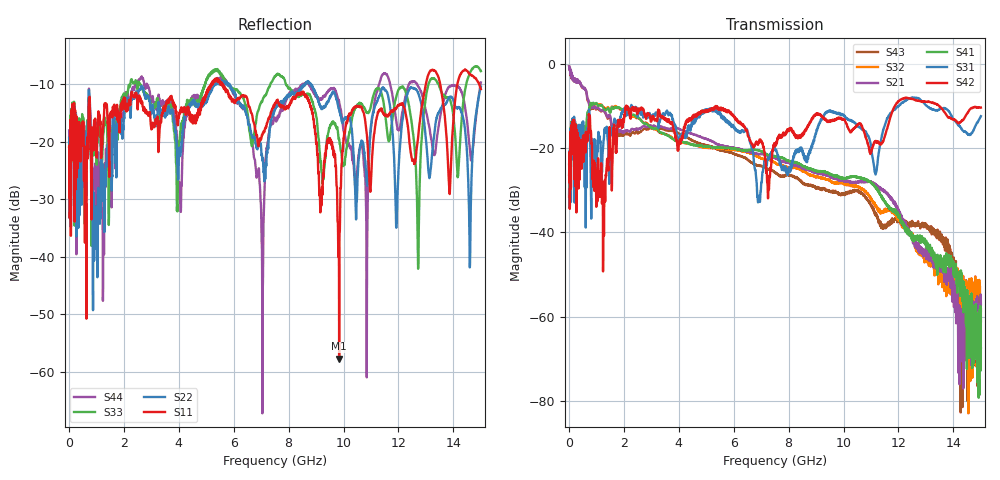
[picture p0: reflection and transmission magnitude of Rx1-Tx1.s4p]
! FILE: N:\QM 2007\Prüfprotokolle\Highspeed\Konfektionierte Ltg\L45593-D106\D30\8216\0002  kpl\IL  mit Chris Boards\Rx1-Tx1.s4p
# MHz S DB R 50.00
! FREQ  S11  S12  S13  S14
!  S21  S22  S23  S24
!  S31  S32  S33  S34
!  S41  S42  S43  S44
!  DB  ANG  DB  ANG  DB  ANG  DB  ANG
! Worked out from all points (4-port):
!   2999 points, 10 MHz to 15 GHz, reference 50 ohm
!   strongest paths, dB at 10 MHz, 3.755 GHz, 7.505 GHz, 11.26 GHz, 15 GHz:
!     S42: -26.3, -13.9, -19.5, -18.6, -10.4
!     S31: -24.0, -12.4, -20.2, -22.3, -12.5
!     S41: -30.9, -17.7, -21.9, -30.1, -67.5
!     S21: -0.7, -15.4, -22.4, -29.1, -57.0
!     S32: -31.6, -17.7, -23.5, -34.7, -58.2
!     S43: -0.6, -16.0, -25.7, -36.9, -61.1
!   lowest |S11| = -57.7 dB at 9.84 GHz (marker M1), VSWR 1.00, Z = 49.9 - j0.0297 ohm
!   |S11| at or under -10 dB: start of sweep to 5.182 GHz; 5.595 GHz to 12.99 GHz (7.399 GHz wide, 79.6 % of centre); 13.52 GHz to 14.14 GHz (619 MHz wide, 4.48 % of centre)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
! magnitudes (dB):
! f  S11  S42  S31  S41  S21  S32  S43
! 10 MHz  -20.8  -26.3  -24.0  -30.9  -0.7  -31.6  -0.6
! 5.615 GHz  -10.2  -10.5  -12.6  -20.0  -19.5  -20.2  -20.7
! 7.045 GHz  -18.8  -18.8  -25.8  -20.9  -21.4  -22.6  -24.4
! 8.5 GHz  -11.6  -16.7  -20.5  -24.2  -24.7  -25.4  -28.2
! 9.84 GHz  -57.7  -13.0  -12.0  -26.9  -27.7  -28.3  -30.8
! 14.6 GHz  -8.2  -10.9  -16.9  -57.6  -58.9  -60.8  -60.7
! 15 GHz  -10.8  -10.4  -12.5  -67.5  -57.0  -58.2  -61.1
